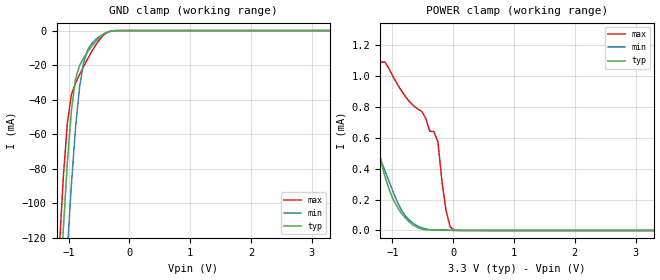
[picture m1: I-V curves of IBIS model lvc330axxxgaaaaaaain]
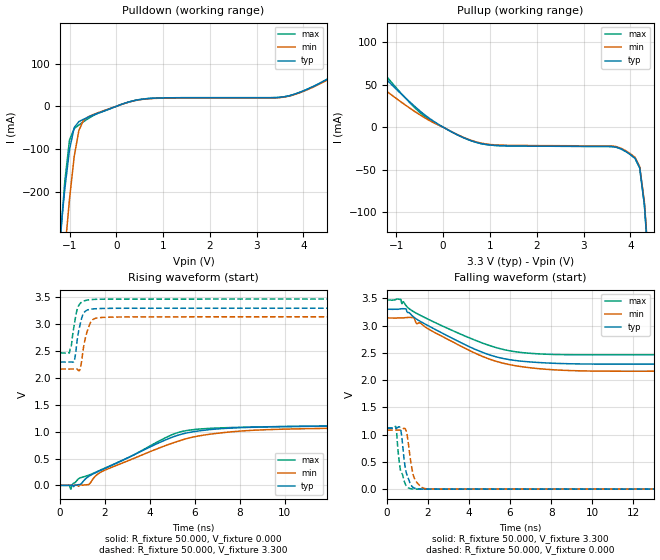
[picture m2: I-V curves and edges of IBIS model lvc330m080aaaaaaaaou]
| IBIS Models Generator: Lattice Radiant Software (64-bit) 2023.2.1.288.0
| Report Generate Date: Jun  5 2024
| Report Generate Time: 12:17:18
| IBIS File LibisMaker.ibs
| Cadence Design Systems, Inc. 2022
[IBIS ver]   4.2
[File Name]   lab03_impl_1.ibs
[File Rev]   1.9
[Date]   Wed Dec 14 00:00:05 PST 2022
[Source]   Lattice Semiconductor 28fdsoi Process
[Notes]   Device: LIFCL-17   Final
   Lattice Semiconductor has worked hard to ensure the
   models below are accurate and complete.  However, the
   data below was generated using simulation of the
   input/output model files for the silicon.  Therefore,
   the data below is for reference and initial design
   purposes only.
   Lattice Semiconductor grants permission to use this
   data for use in printed circuit design using this
   Lattice programmable logic device.  Other use of this
   code, including the selling or duplication of any
   portion is strictly prohibited.
|   NAMING CONVENTION
   The IBIS [Model] header is limited by the specification to a
   total of characters.  With such a set of characters available
   for naming models it becomes important to attempt to
   meaningfully encode the IO standards so they fit within the
   twenty character limit.  It would seem that twenty characters
   would provide room enough for describing IO's.  However, the
   PLD IO structure continues to grow more and more complex.  The
   complexity is making the twenty characters insuffiently
   descriptive.  In order to overcome this issue the naming
   convention described below is implemented to resolve the issue.
The twenty character space is managed as follows:
   bbbvvvsdddprttmaoixx
   b = standard
   v = voltage (x.xx V)
   s = slew code
   d = drive (xx.x ma)
   p = pullmode code
   r = impedance
   t = termination code
   m = mipi hard dphy mode
   o = diff resistor code
   i = diff  current code
   x = reserved
   standard
   LVCMOS   lvc
   LVCMOSH   lvh
   LVCMOSR   lvr
   LVCMOSD   lvd
   LVTTL   lvt
   lvttld   ltd
   sstl_I   ss1
   sstl_II   ss2
   sstld_I   s1d
   sstld_II   s2d
   hsul   hs1
   hsuld   h1d
   hstl_I   hs1
   hstld_I   h1d
   lvds   lvs
   lvdse   lve
   SUBLVDS   slv
   sublvdse   sle
   sublvdseh   slh
   slvs   svs
   mipi   mip
   vref1   vr1
   slew
   na   a
   fast   f
   slow   s
   med   m
   drive
   2   020
   4   040
   6   060
   8   080
   10   100
   12   120
   16   160
   50rs   r50
   na   xxx
   pullmode/clamp on
   none   a/e
   failsafe   a/e
   up   b/f
   down   c/g
   keeper   d/h
   i3c   i
   impedance
   off   a
   termination
   off   aa
   40   bb
   50   cc
   60   dd
   75   ee
   150   ff
   mipi hard dphy mode
   off   a
   lp   l
   hs   h
   differential resistor
   off   a
   100   b
   differential current
   NA   a
   2.0   b
   3.5   c
   Reserved   IO type
   in   input only (mipi: rx)
   ou   output (mipi: tx)
   io   I/O
   od   Open drain
   on   Inverting differential I/O
   op   Non-Inverting differential I/O
   All the IO models are generated with pull mode set to none.
   Lattice Semiconductor Corporation
   5555 NE Moore Court
   Hillsboro, OR 97214
   U.S.A
   TEL: 1-800-Lattice (USA and Canada)
   408-826-6000 (other locations)
   web: http://www.latticesemi.com/
   email: techsupport@latticesemi.com
[Disclaimer] This IBIS source code is intended as a design reference
   which illustrates how the Lattice Semiconductor device operates.
   It is the user's responsibility to verify their design for
   consistency and functionality through the use of formal
   verification methods.  Lattice Semiconductor provides no warranty
   regarding the use or functionality of this data.
[Copyright]   Copyright 2022 by Lattice Semiconductor Corporation
|   Component LIFCL
[Component] LIFCL
[Manufacturer] Lattice Semiconductor Corp.
[Package]
|QFN72
| variable   typ   min   max
R_pkg   0.51641   0.3775   0.86063
L_pkg   2.332e-9   1.653e-9   4.001e-9
C_pkg   3.959e-13   3.388e-13   4.752e-13
[Pin]  signal_name   model_name   R_pin   L_pin   C_pin
57   out2[5]   lvc330m080aaaaaaaaou
51   out2[6]   lvc330m080aaaaaaaaou
44   out2[7]   lvc330m080aaaaaaaaou
42   out2[4]   lvc330m080aaaaaaaaou
43   out2[3]   lvc330m080aaaaaaaaou
55   out2[2]   lvc330m080aaaaaaaaou
53   out2[1]   lvc330m080aaaaaaaaou
52   out2[0]   lvc330m080aaaaaaaaou
59   Clk   lvc330axxxgaaaaaaain
56   En1   lvc330axxxgaaaaaaain
| Models and submodels in the file (2): lvc330axxxgaaaaaaain (Input), lvc330m080aaaaaaaaou (Output)
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[Model] lvc330axxxgaaaaaaain
Model_type Input
Polarity   Non-Inverting
Enable   Active-High
Vinl =  0.800V
Vinh =  2.000V
C_comp   5.000pF   4.000pF   5.500pF
[Temperature Range]   25.000   0.125k   -40.000
[Voltage Range]   3.300V   3.140V   3.470V
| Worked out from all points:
|   GND clamp passes 1 mA (typ) near -0.37 V on its own axis
|   POWER clamp passes 1 mA (typ) near -1.47 V on its own axis
[GND_clamp]
|Voltage   I(typ)   I(min)   I(max)
-3.3V     -1.865A    -1.847A    -1.883A
-1.156V   -160.1mA   -214.1mA   -127.6mA
-1.089V   -115.7mA   -169.6mA   -85.35mA
-1.022V   -76.45mA   -127.5mA   -53.7mA
-955mV    -46.24mA   -89.13mA   -37.05mA
-888mV    -28.3mA    -56.66mA   -30.41mA
-821mV    -20.19mA   -32.82mA   -25.49mA
-754mV    -15.89mA   -18.49mA   -20.81mA
-620mV    -9.094mA   -7.515mA   -12.09mA
-419mV    -1.868mA   -1.846mA   -2.383mA
-218mV    -16.48uA   -78.61uA   -6.639uA
3.3V      0A         0A         0A
[POWER_clamp]
|Voltage   I(typ)   I(min)   I(max)
-3.3V     37.53mA    9.364mA    73.7mA
-1.792V   1.823mA    1.318mA    2.466mA
-1.591V   1.29mA     991.8uA    1.714mA
-1.457V   981.8uA    795.4uA    1.299mA
-1.39V    843.7uA    703.6uA    1.091mA
-1.122V   347.7uA    385.2uA    1.091mA
-854mV    112.9uA    134.5uA    907uA
-586mV    19.15uA    28.85uA    788.2uA
-251mV    3.861uA    1.254uA    573.3uA
-117mV    3.861uA    1.254uA    126.7uA
17mV      69.96nA    1.254uA    1.636uA
3.3V      0A         0A         0A
[Model] lvc330m080aaaaaaaaou
Model_type Output
Polarity   Non-Inverting
Enable   Active-High
Vmeas =  1.650V
Cref =  0.0F
Rref =  1.000M
Vref =  0.0V
C_comp   5.000pF   4.000pF   5.500pF
[Temperature Range]   25.000   0.125k   -40.000
[Voltage Range]   3.300V   3.140V   3.470V
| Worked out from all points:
|   slope of the pulldown table from 0 to 0.495 V, typ, clamps not added: 31.5 ohm
|   slope of the pullup table from 0 to 0.495 V, typ, clamps not added: 35.9 ohm
|   rising waveform, R_fixture 50.000, V_fixture 0.000: 20-80 % time 3.47ns typ, 3.91ns min, 3.27ns max; typ from 0 V to 1.12 V
|   rising waveform, R_fixture 50.000, V_fixture 3.300: 20-80 % time 248ps typ, 295ps min, 236ps max; typ from 2.3 V to 3.3 V
|   falling waveform, R_fixture 50.000, V_fixture 3.300: 20-80 % time 3.22ns typ, 3.2ns min, 3.51ns max; typ from 3.3 V to 2.3 V
|   falling waveform, R_fixture 50.000, V_fixture 0.000: 20-80 % time 273ps typ, 284ps min, 288ps max; typ from 1.12 V to 0 V
[Pulldown]
|Voltage   I(typ)   I(min)   I(max)
-3.3V     -3.025A    -3.614A    -3.918A
-1.2V     -304.3mA   -472.8mA   -317.2mA
-1.1V     -192.9mA   -339.3mA   -175.3mA
-1V       -101.2mA   -217mA     -78.95mA
-900mV    -49.86mA   -117.7mA   -52.21mA
-800mV    -35.81mA   -56.74mA   -43.74mA
-500mV    -20.71mA   -19.77mA   -22.12mA
600mV     17.27mA    16.75mA    17.27mA
3.7V      24.69mA    23.95mA    24.69mA
5.3V      109.4mA    106.1mA    109.4mA
6.1V      131.6mA    127.7mA    131.6mA
6.6V      184.5mA    179mA      184.5mA
[Pullup]
|Voltage   I(typ)   I(min)   I(max)
-3.3V     145.5mA    90.7mA     185.8mA
-3V       114.9mA    81.5mA     156.2mA
-2.7V     96.8mA     74.7mA     125.4mA
-2.4V     95.1mA     71.05mA    105.4mA
-1.9V     90.5mA     66.84mA    102.4mA
-500mV    19.13mA    14.57mA    17.21mA
600mV     -16.01mA   -15.53mA   -16.01mA
3.8V      -25.54mA   -24.77mA   -25.54mA
4.2V      -47.87mA   -46.43mA   -47.87mA
4.3V      -90.8mA    -88.1mA    -90.8mA
4.4V      -169.3mA   -164.2mA   -169.3mA
6.6V      -2.624A    -2.545A    -2.624A
[Ramp]
| variable   typ   min   max
dV/dt_r   0.789/3.474n   0.590/3.936n   0.521/3.276n
dV/dt_f   0.706/3.253n   0.547/3.212n   0.513/3.516n
R_load = 50.000
[Rising Waveform]
R_fixture = 50.000
V_fixture = 0.000
V_fixture_min = 0.000
V_fixture_max = 0.000
|  time   V(typ)   V(min)   V(max)
0s        488.9uV    1.443mV    488.9uV
395ps     637.6uV    952.2uV    3.901mV
475ps     718.1uV    1.451mV    -70.63mV
816ps     13.72mV    -15.69mV   120.4mV
1.256ns   162.7mV    14.22mV    187.3mV
2.016ns   319.3mV    288.2mV    325.9mV
4.885ns   878.7mV    769.5mV    924.9mV
5.78ns    987.4mV    886.1mV    1.03V
9.109ns   1.088V     1.036V     1.091V
20ns      1.119V     1.084V     1.122V
[Rising Waveform]
R_fixture = 50.000
V_fixture = 3.300
V_fixture_min = 3.140
V_fixture_max = 3.470
|  time   V(typ)   V(min)   V(max)
0s        2.297V     2.167V     2.467V
409ps     2.297V     2.166V     2.466V
616ps     2.299V     2.168V     2.961V
734ps     2.622V     2.168V     3.237V
866ps     2.953V     2.141V     3.375V
1.036ns   3.197V     2.555V     3.43V
1.276ns   3.274V     2.953V     3.455V
1.486ns   3.287V     3.096V     3.463V
2.077ns   3.297V     3.131V     3.469V
20ns      3.3V       3.14V      3.47V
[Falling Waveform]
R_fixture = 50.000
V_fixture = 3.300
V_fixture_min = 3.140
V_fixture_max = 3.470
|  time   V(typ)   V(min)   V(max)
0s        3.3V       3.14V      3.47V
666ps     3.307V     3.141V     3.481V
726ps     3.309V     3.14V      3.403V
924ps     3.306V     3.147V     3.369V
1.275ns   3.165V     3.146V     3.261V
1.436ns   3.12V      3.04V      3.227V
4.236ns   2.575V     2.505V     2.741V
6.39ns    2.354V     2.256V     2.514V
9.897ns   2.295V     2.167V     2.465V
20ns      2.297V     2.167V     2.467V
[Falling Waveform]
R_fixture = 50.000
V_fixture = 0.000
V_fixture_min = 0.000
V_fixture_max = 0.000
|  time   V(typ)   V(min)   V(max)
0s        1.119V     1.084V     1.122V
432ps     1.119V     1.083V     1.146V
635ps     1.128V     1.083V     395.6mV
704ps     1.006V     1.09V      298.1mV
846ps     510.1mV    1.117V     138.5mV
936ps     308.8mV    1.065V     61.56mV
1.193ns   62.15mV    421.9mV    5.671mV
1.432ns   8.25mV     133.1mV    217.4uV
1.966ns   398.9uV    4.682mV    -527.1uV
20ns      488.9uV    1.443mV    488.9uV
